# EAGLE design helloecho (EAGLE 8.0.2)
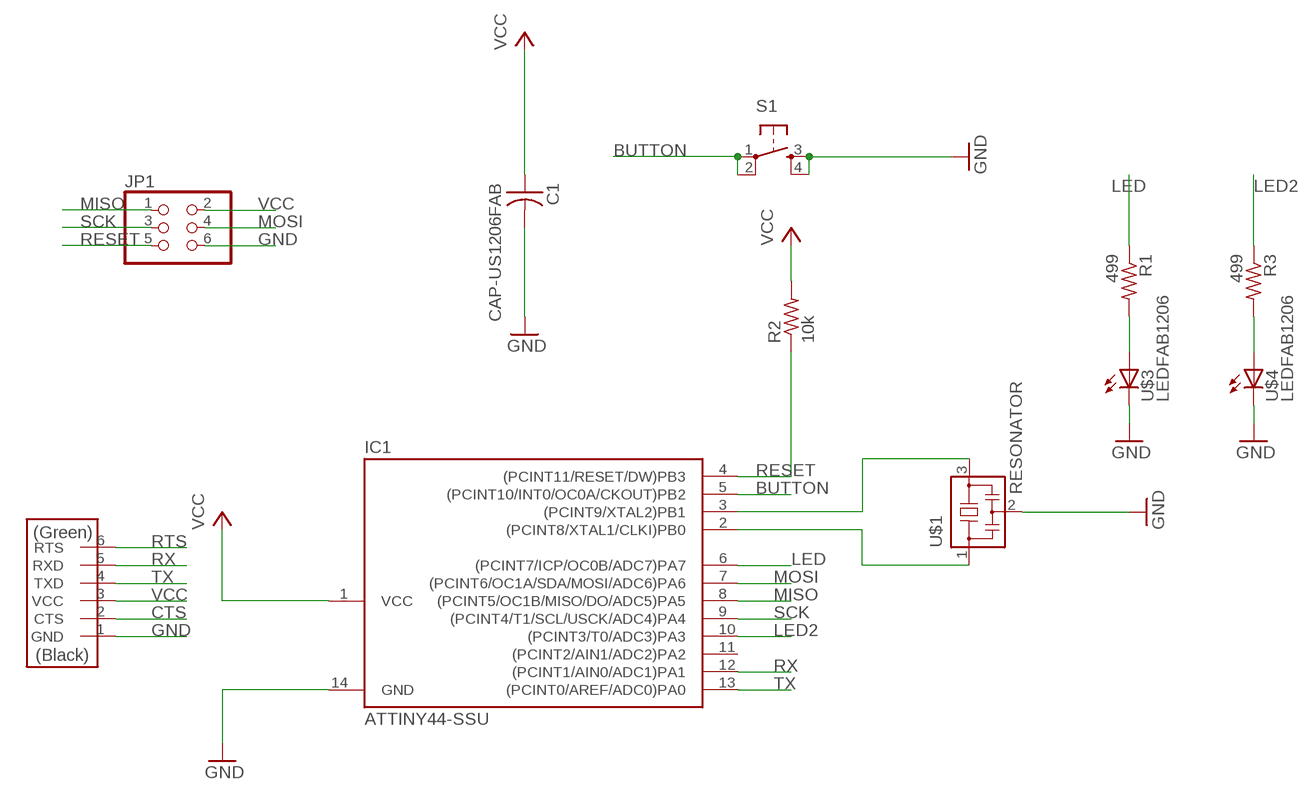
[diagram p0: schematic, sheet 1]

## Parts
C1  CAP-US1206FAB  [C1206FAB]
IC1  ATTINY44-SSU  [SOIC14]
JP1  PINHD-2X3-SMD  [2X03SMD]
R1  499  RES-US1206FAB  [R1206FAB]
R2  10k  RES-US1206FAB  [R1206FAB]
R3  499  RES-US1206FAB  [R1206FAB]
S1  6MM_SWITCH6MM_SWITCH  [6MM_SWITCH]
U$1  RESONATOR  [EFOBM]
U$2  FTDI-SMD-HEADER  [1X06SMD]
U$3  LEDFAB1206  [LED1206FAB]
U$4  LEDFAB1206  [LED1206FAB]

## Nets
BUTTON: IC1.5((PCINT10/INT0/OC0A/CKOUT)PB2) S1.1(P) S1.2(P1)
CTS: U$2.2(CTS)
GND: C1.2 IC1.14(GND) JP1.6 S1.3(S) S1.4(S1) U$1.2 U$2.1(GND) U$3.2(C) U$4.2(C)
LED: IC1.6((PCINT7/ICP/OC0B/ADC7)PA7) R1.1
LED2: IC1.10((PCINT3/T0/ADC3)PA3) R3.1
MISO: IC1.8((PCINT5/OC1B/MISO/DO/ADC5)PA5) JP1.1
MOSI: IC1.7((PCINT6/OC1A/SDA/MOSI/ADC6)PA6) JP1.4
N$2: R1.2 U$3.1(A)
N$3: R3.2 U$4.1(A)
N$4: IC1.2((PCINT8/XTAL1/CLKI)PB0) U$1.1
N$5: IC1.3((PCINT9/XTAL2)PB1) U$1.3
RESET: IC1.4((PCINT11/RESET/DW)PB3) JP1.5 R2.1
RTS: U$2.6(RTS)
RX: IC1.12((PCINT1/AIN0/ADC1)PA1) U$2.5(RXD)
SCK: IC1.9((PCINT4/T1/SCL/USCK/ADC4)PA4) JP1.3
TX: IC1.13((PCINT0/AREF/ADC0)PA0) U$2.4(TXD)
VCC: C1.1 IC1.1(VCC) JP1.2 R2.2 U$2.3(VCC)
Unconnected: IC1.11((PCINT2/AIN1/ADC2)PA2)

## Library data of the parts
C1 = 01_fab:CAP-US
IC1 = 01_fab:ATTINY44
JP1 = 01_fab:PINHD-2X3-SMD: PIN HEADER
R1-R3 = 01_fab:RES-US: Resistor (US Symbol)
S1 = 01_fab:6MM_SWITCH: OMRON SWITCH
U$1 = 01_fab:RESONATOR
U$2 = 01_fab:FTDI-SMD-HEADER
U$3 U$4 = 01_fab:LED: LED

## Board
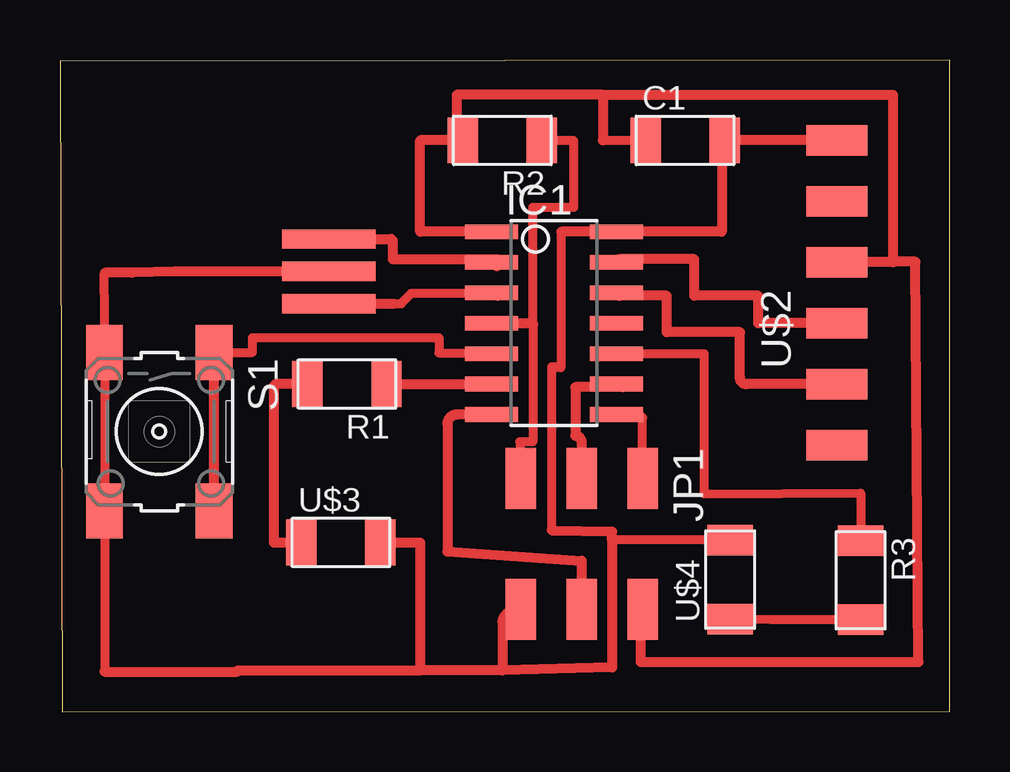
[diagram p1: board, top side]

Size 37.09 x 27.18 mm. Coordinates in mm from the lower left corner, seen from the top.
Outline: 0.1,0 37.09,0.03 37.09,27.18 0,27.13 0.1,0
Copper layers (1*16): Top 0.035mm / dielectric 1.5mm / Bottom 0.035mm
Design rules "modela *": minimum track width 15mil, minimum drill 0.79mm, track to track 0.3985mm, track to pad 0.3985mm, pad to pad 0.3985mm, via to via 0.3985mm, smd to smd 0.3985mm, copper to edge 40mil, drill to drill 8mil, minimum pad ring 10mil, minimum via ring 8mil, stop-mask expansion 4mil, vias tented up to drill 0mil, thermal gap 10mil

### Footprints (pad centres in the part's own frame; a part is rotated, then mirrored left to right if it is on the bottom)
C1206FAB = smd 1.27 x 1.905: 1 -1.651,0; 2 1.651,0
SOIC14 = smd 0.61 x 2.21: 1 -3.81,-2.603; 2 -2.54,-2.603; 3 -1.27,-2.603; 4 0,-2.603; 5 1.27,-2.603; 6 2.54,-2.603; 7 3.81,-2.603; 8 3.81,2.603; 9 2.54,2.603; 10 1.27,2.603; 11 0,2.603; 12 -1.27,2.603; 13 -2.54,2.603; 14 -3.81,2.603
2X03SMD = smd 2.54 x 1.27: 1 -2.54,2.54; 2 2.92,2.54; 3 -2.54,0; 4 2.92,0; 5 -2.54,-2.54; 6 2.92,-2.54
R1206FAB = smd 1.27 x 1.905: 1 -1.651,0; 2 1.651,0
6MM_SWITCH = smd 2.286 x 1.524: 1 -3.302,2.286; 2 3.302,2.286; 3 -3.302,-2.286; 4 3.302,-2.286
EFOBM = smd 0.8 x 3.9: 1 -1.35,0; 2 0,0; 3 1.35,0
1X06SMD = smd 2.54 x 1.27: 1 0,6.35; 2 0,3.81; 3 0,1.27; 4 0,-1.27; 5 0,-3.81; 6 0,-6.35
LED1206FAB = smd 1.27 x 1.905: 1 -1.651,0; 2 1.651,0

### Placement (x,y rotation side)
C1  26.06,23.83 0 top
IC1  20.6,16.21 270 top
JP1  21.74,7.19 270 top
R1  11.96,13.67 180 top
R2  18.44,23.83 180 top
R3  33.38,5.49 270 top
S1  4.14,11.68 270 top
U$1  11.2,18.36 270 top
U$2  32.39,17.48 0 top
U$3  11.71,7.06 0 top
U$4  27.94,5.51 90 top

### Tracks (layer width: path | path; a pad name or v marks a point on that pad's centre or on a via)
BUTTON
  Top 0.381: S1.1 8.03,14.99 8.03,15.6 15.8,15.6 15.8,14.96 18,14.96 IC1.5
  Top 0.406: S1.2 S1.1
GND
  Top 0.381: 20.9,20.02 20.88,20.02 20.88,14.35 20.65,14.35 20.65,14.38 20.5,14.38 20.5,7.57 | 1.88,18.31 1.83,18.21 S1.3 S1.4 1.85,1.68 | U$4.2 23.01,7.16 23.01,7.14
  Top 0.406: 15.01,1.73 7.39,1.73 7.39,1.68 1.85,1.68 | 18.44,1.73 15.01,1.73 | 18.44,1.73 23.01,1.85 23.01,7.14 23.01,7.52 20.5,7.57 | U$3.2 15.01,7.06 15.01,1.73 | JP1.6 arc90 18.44,3.76 18.44,1.73 | U$2.1 C1.2 arc90 27.58,23.7 27.58,20.02 IC1.14 20.9,20.02 | 1.88,18.31 3,18.31 4.8,18.36 U$1.2
LED
  Top 0.406: R1.1 IC1.6
LED2
  Top 0.381: IC1.10 26.85,14.94 26.85,9.09 33.38,9.12 R3.1
MISO
  Top 0.381: JP1.1 24.28,12.27 24.21,12.34 23.25,12.34 IC1.8
MOSI
  Top 0.406: IC1.7 16.54,12.4 arc90 16.15,12.01 16.15,6.68 21.74,6.3 JP1.4
N$2
  Top 0.406: R1.2 9.04,13.67 arc90 8.92,13.54 8.92,7.06 U$3.1
N$3
  Top 0.381: R3.2 29.64,3.84 U$4.1
N$4
  Top 0.406: 18.2,18.57 arc90 IC1.2 arc90 18.25,18.87 13.87,18.87 13.87,19.63 arc90 13.79,19.71 U$1.1
N$5
  Top 0.381: 13.92,17.01 14.22,17.01 14.66,17.45 17.97,17.45 IC1.3
  Top 0.406: U$1.3 13.92,17.01 | IC1.3 arc-90 18.25,17.35
RESET
  Top 0.381: R2.1 21.39,23.83 21.39,23.8 21.41,23.8 21.41,21.03 19.71,21.03 19.71,16.1 19.71,11.25 19.18,11.25 19.18,10.77 19.2,10.77 JP1.5
  Top 0.406: IC1.4 19.71,16.21 19.71,16.1
RX
  Top 0.406: U$2.5 28.6,13.67 arc-90 28.35,13.92 28.35,15.82 25.3,15.82 25.3,17.35 23.33,17.35 arc-90 IC1.12
SCK
  Top 0.406: IC1.9 arc-90 23.46,13.54 21.49,13.54 21.49,11.51 arc-90 21.74,11.25 JP1.3
TX
  Top 0.406: U$2.4 29.11,16.21 29.11,17.35 26.44,17.35 26.44,18.87 23.33,18.87 arc90 IC1.13
VCC
  Top 0.381: 22.63,23.83 C1.1
  Top 0.406: IC1.1 15.01,20.02 15.01,23.83 16.54,23.83 | 16.54,23.83 R2.2 | U$2.3 34.72,18.75 34.72,18.77 | 22.63,25.73 22.63,23.83 | 22.63,25.73 34.72,25.73 34.72,18.77 | 22.63,25.73 16.54,25.73 16.54,23.83 | JP1.2 24.21,4.27 24.21,2.08 35.79,2.08 35.66,18.77 34.72,18.77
